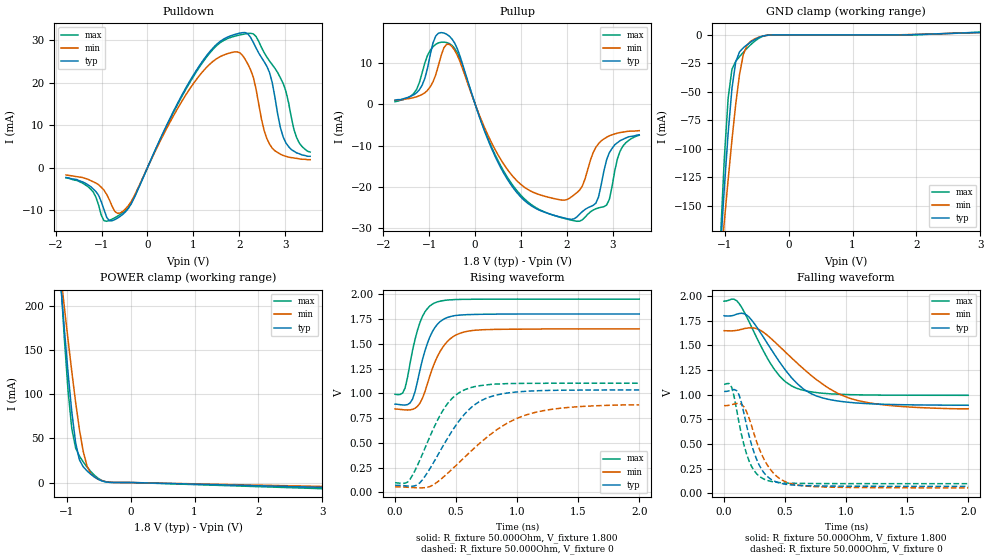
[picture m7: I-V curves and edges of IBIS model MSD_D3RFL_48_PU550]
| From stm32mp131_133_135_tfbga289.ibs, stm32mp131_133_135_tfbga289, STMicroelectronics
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[Model] MSD_D3RFL_48_PU550
Model_type   I/O
C_comp 2.403pF   2.320pF   2.527pF
Vinh = 1.440V
Vinl = 360.000mV
Vmeas = 900.000mV
Vref = 900.000mV
[Model Spec]
Vinh   1.440V   1.365V   1.515V
Vinl   360.000mV   285.000mV   435.000mV
Vmeas   900.000mV   825.000mV   975.000mV
Vref   900.000mV   825.000mV   975.000mV
[Temperature Range]   25.000   125.000   -40.000
[Voltage Range]   1.800V   1.650V   1.950V
[GND Clamp Reference]   0.00V   0.00V   0.00V
[Pulldown Reference]   0.00V   0.00V   0.00V
[POWER Clamp Reference]   1.800V   1.650V   1.950V
[Pullup Reference]   1.800V   1.650V   1.950V
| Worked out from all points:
|   slope of the pulldown table from 0 to 0.27 V, typ, clamps not added: 41 ohm
|   slope of the pullup table from 0 to 0.27 V, typ, clamps not added: 32.3 ohm
|   GND clamp passes 1 mA (typ) near -0.40 V on its own axis
|   POWER clamp passes 1 mA (typ) near -0.41 V on its own axis
|   rising waveform, R_fixture 50.000Ohm, V_fixture 1.800: 20-80 % time 130ps typ, 164ps min, 113ps max; typ from 0.891 V to 1.8 V
|   rising waveform, R_fixture 50.000Ohm, V_fixture 0: 20-80 % time 313ps typ, 494ps min, 240ps max; typ from 0.072 V to 1.03 V
|   falling waveform, R_fixture 50.000Ohm, V_fixture 1.800: 20-80 % time 331ps typ, 476ps min, 261ps max; typ from 1.8 V to 0.893 V
|   falling waveform, R_fixture 50.000Ohm, V_fixture 0: 20-80 % time 141ps typ, 177ps min, 121ps max; typ from 1.03 V to 0.071 V
[GND Clamp]
-1.773V   -890.2mA   -681.4mA   -1.194A
-1.064V   -187.1mA   -201.7mA   -177.2mA
-1.005V   -134.3mA   -163.8mA   -108.3mA
-945.5mV  -86.36mA   -127.2mA   -55.56mA
-886.4mV  -47.34mA   -92.5mA    -30.23mA
-827.3mV  -23.67mA   -61.01mA   -23.24mA
-768.2mV  -14.92mA   -34.96mA   -19.11mA
-709.1mV  -11.32mA   -17.42mA   -15.31mA
-650mV    -8.623mA   -8.965mA   -11.75mA
-531.8mV  -4.14mA    -3.5mA     -5.545mA
-295.4mV  -89.22uA   -144.4uA   -78.82uA
3.545V    3.247mA    2.865mA    3.764mA
[Power Clamp]
-1.745V   860mA      674.5mA    1.126A
-1.095V   228.4mA    237.9mA    233.1mA
-1.036V   174.8mA    199.6mA    164.1mA
-977.3mV  124.4mA    161.9mA    103.9mA
-918.2mV  79.71mA    125.5mA    60.63mA
-859.1mV  45.09mA    91.13mA    39.12mA
-800mV    25.81mA    60.25mA    30.04mA
-740.9mV  17.95mA    35.4mA     23.48mA
-681.8mV  13.25mA    19.01mA    17.68mA
-504.5mV  3.57mA     3.681mA    4.679mA
-327.3mV  155.3uA    337.8uA    197uA
3.573V    -6.594mA   -5.322mA   -8.376mA
[Pulldown]
-1.773V   -2.3mA     -1.7mA     -2.4mA
-1.182V   -5mA       -3.3mA     -5.7mA
-945.5mV  -9.87mA    -5.3mA     -12.49mA
-531.8mV  -10.94mA   -10.23mA   -10.53mA
1.064V    22.92mA    20.75mA    22.58mA
2.068V    31.83mA    26.53mA    31.41mA
2.305V    29.56mA    21.37mA    31.55mA
2.541V    25.01mA    8.8mA      27.15mA
2.718V    20.08mA    4.6mA      24.29mA
3.014V    5.9mA      2.7mA      18.1mA
3.25V     3.5mA      2.2mA      7.1mA
3.545V    2.7mA      1.9mA      3.7mA
[Pullup]
-1.745V   1mA        953.9uA    600uA
-1.332V   2.3mA      1.608mA    2.669mA
-1.036V   8.8mA      3.377mA    11.85mA
-859.1mV  16.48mA    7.104mA    14.48mA
-622.7mV  16.92mA    14.48mA    14.91mA
-386.4mV  13.35mA    11.77mA    12.33mA
795.5mV   -19.73mA   -17.13mA   -19.24mA
2.214V    -27.27mA   -21.4mA    -28.32mA
2.745V    -19.47mA   -8.877mA   -24.92mA
2.923V    -11.7mA    -7.638mA   -23mA
3.041V    -9.8mA     -7.192mA   -16.09mA
3.573V    -7.4mA     -6.4mA     -7.508mA
[Ramp]
R_load=50.000Ohm
dV/dt_r   561.336mV/222.000ps  489.975mV/329.500ps  587.976mV/177.500ps
dV/dt_f   561.150mV/237.000ps  488.094mV/326.500ps  587.976mV/191.000ps
[Rising waveform]
R_fixture=50.000Ohm
V_fixture=1.800
V_fixture_min=1.650
V_fixture_max=1.950
0s        891.3mV    842.9mV    990.3mV
62ps      882.5mV    835.1mV    1.003V
82ps      881.8mV    832.7mV    1.053V
143ps     941.6mV    838.3mV    1.432V
225ps     1.342V     952.5mV    1.777V
266ps     1.508V     1.1V       1.856V
327ps     1.665V     1.317V     1.913V
450ps     1.773V     1.548V     1.943V
613ps     1.794V     1.63V      1.948V
2ns       1.8V       1.65V      1.95V
[Rising waveform]
R_fixture=50.000Ohm
V_fixture=0
0s        72.2mV     56.33mV    98.29mV
103ps     65.08mV    52.93mV    105.1mV
205ps     100.2mV    46.69mV    332.1mV
286ps     241.3mV    60.49mV    565.2mV
409ps     502.9mV    169.7mV    859.5mV
572ps     793.2mV    357.9mV    1.037V
776ps     963.4mV    580.4mV    1.089V
1.062ns   1.02V      777.7mV    1.101V
1.409ns   1.032V     856.5mV    1.102V
2ns       1.034V     883.5mV    1.102V
[Falling waveform]
R_fixture=50.000Ohm
V_fixture=1.800
V_fixture_min=1.650
V_fixture_max=1.950
0s        1.8V       1.649V     1.948V
103ps     1.816V     1.652V     1.953V
205ps     1.787V     1.678V     1.739V
286ps     1.652V     1.661V     1.531V
409ps     1.416V     1.542V     1.262V
491ps     1.269V     1.446V     1.144V
593ps     1.12V      1.327V     1.066V
756ps     987.4mV    1.153V     1.022V
1.083ns   916.5mV    944.8mV    999.4mV
2ns       893.2mV    857.2mV    994.2mV
[Falling waveform]
R_fixture=50.000Ohm
V_fixture=0
0s        1.033V     888.7mV    1.105V
62ps      1.048V     898.6mV    1.076V
123ps     997.3mV    912.2mV    712.3mV
164ps     802.6mV    874.7mV    486.7mV
205ps     582.7mV    761.4mV    327.6mV
266ps     346.6mV    525.2mV    199.2mV
327ps     207.7mV    346.6mV    144.2mV
450ps     106.6mV    154.3mV    109.6mV
613ps     80.47mV    82.05mV    101.3mV
2ns       71.25mV    55.72mV    98.18mV
